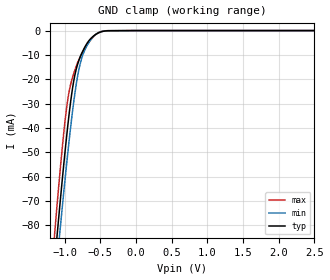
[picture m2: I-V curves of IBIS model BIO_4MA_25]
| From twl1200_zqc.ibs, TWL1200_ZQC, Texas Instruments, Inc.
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[Model]   BIO_4MA_25
Model_type  Input
Vinl=0.875
Vinh=1.625
| variable   typ   min   max
C_comp   2.78pF   2.35pF   3.44pF
[Temperature Range]   40   100   -40
| Ambient temperature   25   85   -40
[Voltage range]   2.5   2.3   2.7
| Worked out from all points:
|   GND clamp passes 1 mA (typ) near -0.53 V on its own axis
[GND Clamp]
| BIO_4MA_25
|   Voltage   I(typ)   I(min)   I(max)
-2.5V     -587.4mA   -575.4mA   -603.8mA
-1.14V    -95.72mA   -105.9mA   -83.71mA
-1.095V   -81.06mA   -91.79mA   -68.33mA
-1.07V    -73.08mA   -84.08mA   -60.07mA
-1.06V    -69.93mA   -81.02mA   -56.84mA
-960mV    -40.49mA   -51.77mA   -29.36mA
-905mV    -27.11mA   -37.25mA   -20.98mA
-855mV    -18.23mA   -25.77mA   -16.19mA
-795mV    -11.92mA   -15.42mA   -11.63mA
-740mV    -8.153mA   -9.687mA   -8.49mA
-535mV    -1.097mA   -993uA     -1.036mA
2.5V      592.1pA    215.9nA    86.51pA
